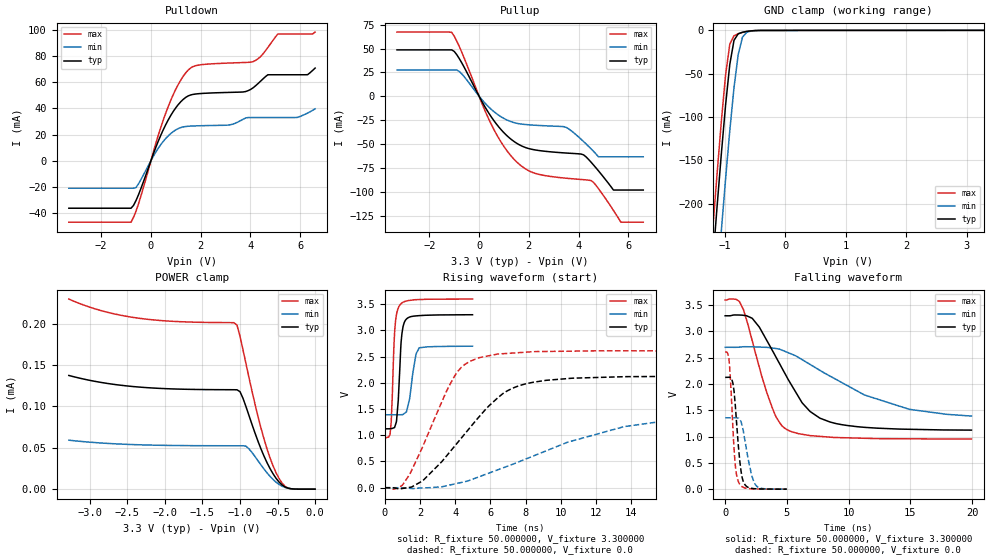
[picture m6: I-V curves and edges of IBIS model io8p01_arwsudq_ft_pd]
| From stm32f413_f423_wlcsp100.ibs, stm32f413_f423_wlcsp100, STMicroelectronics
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|   Model io8p01_arwsudq_ft_pd
[Model]  io8p01_arwsudq_ft_pd
Model_type I/O
Polarity   Non-Inverting
Enable   Active-Low
Vinl =   0.990000V
Vinh =   2.310000V
Vmeas =  1.650000V
Cref =   50.000000pF
Rref =   100.000000M
Vref =   0.0V
C_comp   2.905500pF   2.823600pF   2.987900pF
[Temperature Range]   25.000000   0.125000k   -40.000000
[Pullup Reference]   3.300000V   2.700000V   3.600000V
[Pulldown Reference]   0.0V   0.0V   0.0V
[POWER Clamp Reference]   3.300000V   2.700000V   3.600000V
[GND Clamp Reference]   0.0V   0.0V   0.0V
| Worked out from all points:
|   slope of the pulldown table from 0 to 0.495 V, typ, clamps not added: 20.9 ohm
|   slope of the pullup table from 0 to 0.495 V, typ, clamps not added: 22.6 ohm
|   GND clamp passes 1 mA (typ) near -0.62 V on its own axis
|   rising waveform, R_fixture 50.000000, V_fixture 3.300000: 20-80 % time 213ps typ, 338ps min, 189ps max; typ from 1.12 V to 3.3 V
|   rising waveform, R_fixture 50.000000, V_fixture 0.0: 20-80 % time 3.35ns typ, 6.88ns min, 2.1ns max; typ from 0 V to 2.13 V
|   falling waveform, R_fixture 50.000000, V_fixture 3.300000: 20-80 % time 3.27ns typ, 6.72ns min, 2.01ns max; typ from 3.3 V to 1.12 V
|   falling waveform, R_fixture 50.000000, V_fixture 0.0: 20-80 % time 460ps typ, 654ps min, 373ps max; typ from 2.13 V to 0 V
[Pulldown]
|Voltage   I(typ)   I(min)   I(max)
-3.3V     -36.4mA    -21.07mA   -47.09mA
-800mV    -36.4mA    -21.07mA   -47.09mA
-600mV    -30.5mA    -20.54mA   -38.69mA
700mV     31.4mA     19.11mA    41.71mA
1.2V      45.15mA    25.37mA    61.75mA
1.6V      50.35mA    26.5mA     71.06mA
3.1V      52.27mA    27.26mA    74.75mA
4.1V      55.71mA    33.04mA    75.8mA
4.7V      65.8mA     33.04mA    86.69mA
5.1V      65.8mA     33.04mA    97.03mA
6.3V      65.87mA    36.5mA     97.03mA
6.6V      70.92mA    39.71mA    98.48mA
[Pullup]
|Voltage   I(typ)   I(min)   I(max)
-3.3V     48.55mA    27.44mA    67.2mA
-1.1V     48.55mA    27.44mA    66.9mA
-700mV    35.13mA    23.48mA    46.33mA
500mV     -22.07mA   -14mA      -30.03mA
1.5V      -49.1mA    -28.3mA    -68.56mA
2.2V      -56.04mA   -30.32mA   -80.35mA
3.5V      -59.53mA   -32.66mA   -85.92mA
4.5V      -69.08mA   -55.13mA   -88.39mA
4.8V      -78.24mA   -63.5mA    -96.88mA
5.4V      -98.3mA    -63.5mA    -119.6mA
5.7V      -98.3mA    -63.5mA    -132mA
6.6V      -98.3mA    -63.5mA    -132mA
[GND_clamp]
|Voltage   I(typ)   I(min)   I(max)
-3.3V     -2.317A    -2.396A    -2.29A
-1.2V     -266mA     -356.3mA   -228.4mA
-1.13V    -203.2mA   -293mA     -165.3mA
-1.06V    -142.7mA   -231.3mA   -105.2mA
-990mV    -86.51mA   -171.7mA   -51.78mA
-920mV    -39.3mA    -115.7mA   -15.95mA
-850mV    -11.38mA   -65.76mA   -6.112mA
-780mV    -3.842mA   -27.55mA   -3.895mA
-710mV    -2.102mA   -7.755mA   -2.396mA
-640mV    -1.159mA   -2.138mA   -1.234mA
-570mV    -535.1uA   -809uA     -490.4uA
3.28V     81.28uA    57.87uA    93.98uA
[POWER_clamp]
|Voltage   I(typ)   I(min)   I(max)
-3.28V    137.3uA    59.14uA    229.6uA
-2.36V    123.4uA    53.65uA    206.6uA
-1.08V    120.1uA    52.41uA    201.1uA
-1.04V    120uA      52.41uA    198uA
-1V       117.7uA    52.4uA     184.5uA
-920mV    99.46uA    51.91uA    151.2uA
-720mV    48.42uA    29.12uA    73.51uA
-600mV    24.82uA    15.47uA    37.72uA
-520mV    13.1uA     8.45uA     19.84uA
-440mV    5.058uA    3.61uA     7.276uA
-360mV    1.193uA    1.129uA    1.311uA
0V        0A         0A         0A
[Ramp]
| variable   typ   min   max
dV/dt_r  1.27680/3.34462n   0.79836/6.88465n   1.56659/2.10027n
dV/dt_f  1.30212/3.27572n   0.74022/6.66065n   1.58738/2.00895n
R_load = 50.000000
[Rising Waveform]
R_fixture= 50.000000
V_fixture= 3.300000
V_fixture_min= 2.700000
V_fixture_max= 3.600000
|time   V(typ)   V(min)   V(max)
0s        1.123V     1.391V     953.9mV
300.3ps   1.125V     1.391V     1.012V
370.4ps   1.127V     1.391V     1.254V
570.6ps   1.158V     1.391V     2.997V
670.7ps   1.27V      1.39V      3.305V
830.8ps   2.083V     1.39V      3.468V
981ps     2.945V     1.393V     3.525V
1.241ns   3.219V     1.454V     3.561V
1.962ns   3.282V     2.668V     3.588V
4.985ns   3.299V     2.699V     3.598V
[Rising Waveform]
R_fixture= 50.000000
V_fixture= 0.0
V_fixture_min= 0.0
V_fixture_max= 0.0
|time   V(typ)   V(min)   V(max)
0s        360.8uV    205.7uV    689.3uV
1.001ns   -14.87mV   -990uV     47.26mV
2.162ns   132.8mV    -2.671mV   786.9mV
3.964ns   789.9mV    71.54mV    2.126V
4.565ns   1.034V     116.5mV    2.354V
5.325ns   1.34V      204.8mV    2.475V
6.767ns   1.808V     385.2mV    2.557V
8.408ns   2.01V      601.3mV    2.594V
13.61ns   2.117V     1.166V     2.611V
19.94ns   2.127V     1.357V     2.611V
[Falling Waveform]
R_fixture= 50.000000
V_fixture= 3.300000
V_fixture_min= 2.700000
V_fixture_max= 3.600000
|time   V(typ)   V(min)   V(max)
0s        3.299V     2.699V     3.598V
920.9ps   3.313V     2.699V     3.607V
1.481ns   3.307V     2.709V     3.415V
2.202ns   3.247V     2.707V     2.813V
3.764ns   2.663V     2.687V     1.579V
5.005ns   2.128V     2.606V     1.133V
6.847ns   1.485V     2.377V     1.02V
8.488ns   1.278V     2.151V     989.5mV
14.89ns   1.139V     1.52V      958.1mV
19.94ns   1.123V     1.391V     953.9mV
[Falling Waveform]
R_fixture= 50.000000
V_fixture= 0.0
V_fixture_min= 0.0
V_fixture_max= 0.0
|time   V(typ)   V(min)   V(max)
0s        2.127V     1.357V     2.611V
300.3ps   2.129V     1.357V     2.481V
620.6ps   2.022V     1.357V     1.196V
820.8ps   1.594V     1.359V     454.5mV
1.091ns   765.9mV    1.351V     131.2mV
1.291ns   332.3mV    1.279V     61.22mV
1.481ns   139mV      1.092V     34.01mV
2.142ns   16.11mV    268.7mV    6.517mV
2.442ns   8.423mV    87.97mV    4.67mV
4.985ns   360.8uV    205.7uV    689.3uV
